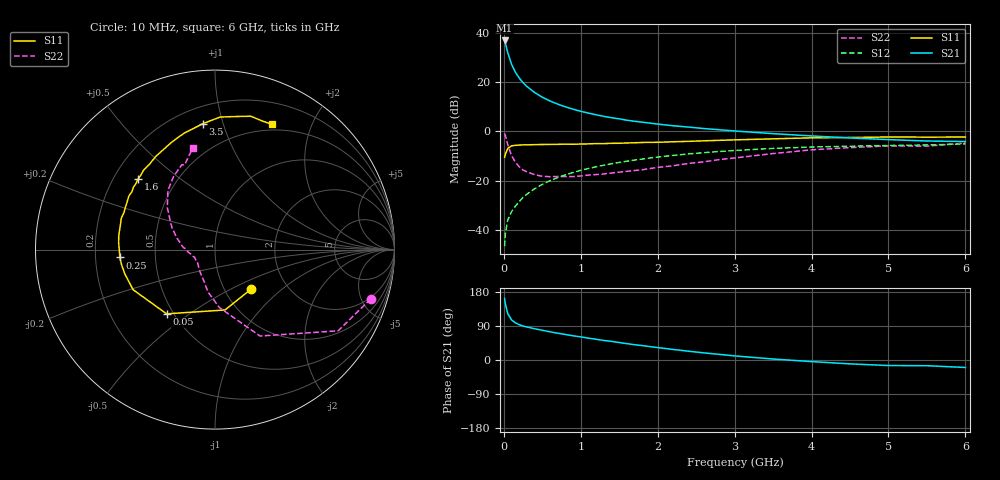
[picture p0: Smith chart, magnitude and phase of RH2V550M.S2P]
! SIEMENS Small Signal Semiconductors
! BFR106
! Si NPN RF Bipolar Junction Transistor in SOT23
! VCE = 2.5 V  IC = 50 mA
! Common Emitter S-Parameters:  August  1996
# GHz  S  MA  R  50
!  f  S11  S21  S12  S22
! GHz  MAG  ANG  MAG  ANG  MAG  ANG  MAG  ANG
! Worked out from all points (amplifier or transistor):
!   36 points, 10 MHz to 6 GHz, reference 50 ohm
!   highest |S21| = 36.9 dB at 10 MHz (marker M1)
!   |S21| within 3 dB of that: start of sweep to 35.48 MHz
!   unconditionally stable (mu >= 1): 232.5 MHz to 2.542 GHz; 5.351 GHz to end of sweep
!   at 250 MHz: K = 1.01, MAG = 22.6 dB, |S12| = -26.8 dB
!   at 1.4 GHz: K = 1.06, MAG = 7.8 dB, |S12| = -13.1 dB
!   at 6 GHz: K = 1.00, MAG = 0.1 dB, |S12| = -5.1 dB
!   S11 on the Smith chart (normalised r, x): 10 MHz: 1.33, -0.64; 50 MHz: 0.46, -0.41; 250 MHz: 0.31, -0.04; 1.6 GHz: 0.30, +0.36; 3.5 GHz: 0.31, +0.86; 6 GHz: 0.43, +1.47
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0.01  0.2983 -47.4  69.65 162.2  0.0047 78.4  0.9098 -17.6
0.02  0.341 -80.6  61.77 148.2  0.0084 66.8  0.822 -33.4
0.05  0.4481 -127.0  39.91 122.7  0.0158 59.4  0.5429 -62.5
0.1  0.5082 -153.9  23.02 105.9  0.0235 60.5  0.3236 -85.7
0.15  0.5203 -164.9  15.81 98.0  0.0305 63.8  0.2385 -99.6
0.2  0.5272 -170.8  12.06 93.3  0.0376 67.6  0.191 -108.0
0.25  0.532 -175.3  9.664 89.7  0.0457 68.9  0.164 -117.0
0.3  0.5322 -178.1  8.109 87.1  0.0534 70.1  0.1513 -123.0
0.4  0.5381 175.9  6.141 82.5  0.0686 71.0  0.1323 -133.6
0.5  0.5418 171.9  4.92 78.4  0.0841 71.0  0.1229 -141.0
0.6  0.5427 167.8  4.128 74.4  0.1001 70.3  0.1203 -145.9
0.7  0.5458 164.5  3.57 70.7  0.1158 69.7  0.1215 -150.6
0.9  0.5476 157.9  2.812 64.0  0.1469 67.1  0.1207 -159.2
1.1  0.5574 151.3  2.342 57.7  0.1767 64.3  0.1299 -164.0
1.3  0.5641 145.1  2.014 51.6  0.2062 61.2  0.1368 -169.9
1.6  0.5813 137.4  1.684 43.1  0.2482 56.5  0.1549 -177.1
2.2  0.615 122.5  1.299 27.9  0.3254 46.6  0.2006 168.1
2.8  0.6571 108.5  1.079 14.9  0.3902 36.8  0.2675 153.3
3.5  0.7047 95.5  0.898 2.6  0.451 26.0  0.3549 138.5
4.5  0.7502 81.2  0.734 -10.2  0.5002 11.7  0.4688 119.4
5.5  0.7634 69.5  0.637 -15.1  0.5292 2.7  0.5011 109.8
6  0.7667 65.4  0.622 -19.7  0.5576 -4.2  0.579 102.4
